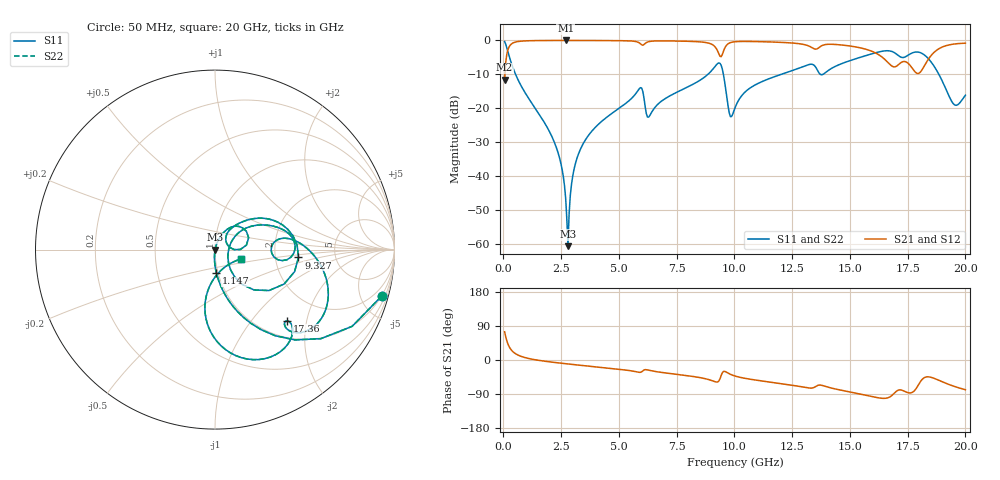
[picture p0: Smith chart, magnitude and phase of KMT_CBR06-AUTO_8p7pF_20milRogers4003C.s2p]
! Data measured by Modelithics Inc. support@modelithics.com 813-866-6335
! KEMET CBR06-AUTO 8.7pF, Pad Width= 0.851mm, Pad Length= 0.64mm, Pad Gap= 0.62mm, 20mil Rogers 4003C substrate Data, January 2022
# hz S ma R 50
! 2 Port Network Data from SP1.SP block
! freq  magS11  angS11  magS21  angS21  magS12  angS12  magS22  angS22
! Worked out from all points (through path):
!   401 points, 50 MHz to 20 GHz, reference 50 ohm
!   highest |S21| = -0.01 dB at 2.693 GHz (marker M1); lowest = -11.5 dB at 50 MHz (marker M2)
!   group delay of S21, straight-line fit = 13.4 ps
!   lowest |S11| = -60.5 dB at 2.793 GHz (marker M3), VSWR 1.00, Z = 50.1 + j0.00847 ohm
!   |S11| at or under -10 dB: 526.5 MHz to 8.847 GHz (8.321 GHz wide, 178 % of centre); 9.523 GHz to 12.01 GHz (2.491 GHz wide, 23.1 % of centre); 18.85 GHz to end of sweep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
!   |S22| runs from -60.5 to -0.3 dB; largest |S21 - S12| = 0
!   S11 on the Smith chart (normalised r, x): 50 MHz: 0.98, -7.18; 1.147 GHz: 0.98, -0.26; 9.327 GHz: 2.71, -0.30; 17.36 GHz: 1.32, -1.54; 20 GHz: 1.34, -0.14
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5e7  0.964 -15.6  0.2654 74.4  0.2654 74.4  0.964 -15.6
3.99125e8  0.4073 -67.4  0.9127 22.5  0.9127 22.5  0.4073 -67.4
1.14725e9  0.1313 -86.5  0.9906 3.2  0.9906 3.2  0.1313 -86.5
2.294375e9  0.02637 -95.3  0.9987 -7.1  0.9987 -7.1  0.02637 -95.3
2.693375e9  0.004787 -89.1  0.999 -9.8  0.999 -9.8  0.004787 -89.1
2.793125e9  0.0009437 5.1  0.999 -10.5  0.999 -10.5  0.0009437 5.1
3.0425e9  0.01212 73.4  0.9989 -12.1  0.9989 -12.1  0.01212 73.4
3.391625e9  0.02771 73.6  0.9985 -14.3  0.9985 -14.3  0.02771 73.6
5.885375e9  0.1956 38.2  0.9181 -32.5  0.9181 -32.5  0.1956 38.2
6.284375e9  0.07446 31.2  0.9585 -27.0  0.9585 -27.0  0.07446 31.2
6.73325e9  0.1194 53.5  0.9829 -31.8  0.9829 -31.8  0.1194 53.5
9.32675e9  0.4672 -5.4  0.6331 -55.4  0.6331 -55.4  0.4672 -5.4
9.8255e9  0.07587 -16.6  0.9285 -37.7  0.9285 -37.7  0.07587 -16.6
1.0025e10  0.1019 25.5  0.9567 -42.3  0.9567 -42.3  0.1019 25.5
1.336662e10  0.4454 0.1  0.7804 -73.9  0.7804 -73.9  0.4454 0.1
1.511225e10  0.519 0.1  0.8174 -85.7  0.8174 -85.7  0.519 0.1
1.670825e10  0.7025 -36.4  0.452 -98.1  0.452 -98.1  0.7025 -36.4
1.735662e10  0.5656 -44.6  0.4902 -82.3  0.4902 -82.3  0.5656 -44.6
1.795512e10  0.6735 -62.7  0.3265 -66.8  0.3265 -66.8  0.6735 -62.7
1.870325e10  0.3883 -97.4  0.6955 -49.8  0.6955 -49.8  0.3883 -97.4
1.950125e10  0.115 -67.4  0.8844 -69.3  0.8844 -69.3  0.115 -67.4
2e10  0.1563 -19.3  0.91 -78.4  0.91 -78.4  0.1563 -19.3
